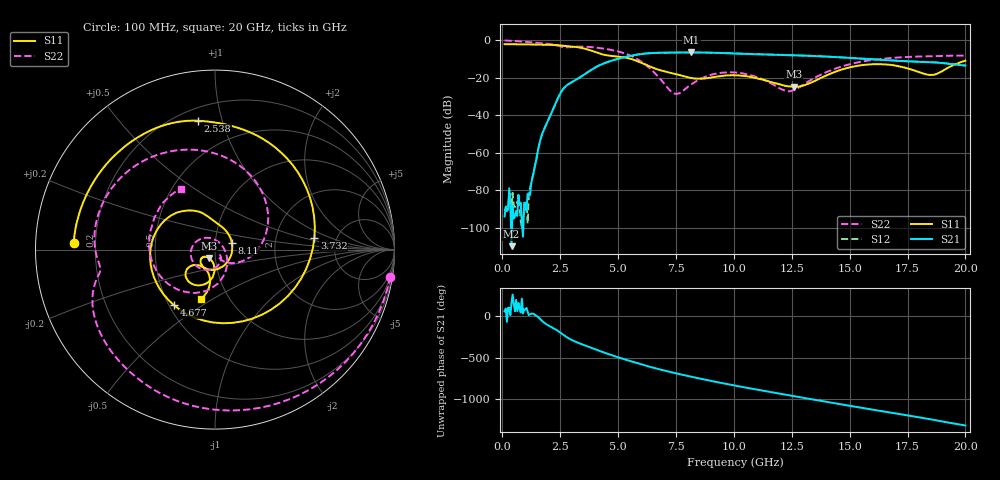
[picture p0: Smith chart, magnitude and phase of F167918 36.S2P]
!  2-Port S-parameters saved by WinCal
! VAR MeasName=S-Parameters (CALIBRATED_DATA) read from VNA (N5242A)
! VAR MeasDate=2016-11-22 10:26:28
! VAR NAME=F167918 36
! VAR FILENAME=F167918 36.S2P
! VAR DATE=2016-11-22 10:26:28
! VAR PHYS_PORTS=1,2
# Hz S DB R 50
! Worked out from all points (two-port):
!   401 points, 100 MHz to 20 GHz, reference 50 ohm
!   highest |S21| = -6.49 dB at 8.159 GHz (marker M1); lowest = -109.7 dB at 398.5 MHz (marker M2)
!   |S21| within 3 dB of the highest: 5.122 GHz to 15.18 GHz (10.06 GHz wide, 99.1 % of centre)
!   lowest |S11| = -24.8 dB at 12.59 GHz (marker M3), VSWR 1.12, Z = 46.6 - j4.41 ohm
!   |S11| at or under -10 dB: 5.578 GHz to end of sweep
!   |S22| runs from -28.6 to -0.1 dB; largest |S21 - S12| = 0.005
!   S11 on the Smith chart (normalised r, x): 100 MHz: 0.12, +0.02; 2.538 GHz: 0.28, +0.84; 3.732 GHz: 3.39, +0.65; 4.677 GHz: 0.53, -0.39; 8.11 GHz: 1.20, +0.09; 20 GHz: 0.74, -0.45
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1e8  -2.07 177.3  -93.89 59.4  -91.08 152.3  -0.10 -8.7
3.985e8  -2.10 169.3  -109.69 158.8  -89.02 177.6  -0.29 -33.0
1.14475e9  -2.23 149.0  -81.51 14.4  -83.80 37.4  -0.96 -87.9
1.74175e9  -2.35 130.4  -49.30 -62.0  -49.34 -62.2  -1.62 -124.9
2.53775e9  -2.80 97.5  -27.63 157.0  -27.63 156.8  -3.42 -166.5
3.43325e9  -4.11 38.5  -19.10 23.2  -19.12 23.2  -3.37 160.8
3.73175e9  -5.07 6.8  -16.65 -8.1  -16.67 -7.9  -3.53 146.4
4.22925e9  -7.19 -61.8  -13.16 -60.5  -13.13 -60.3  -4.18 121.4
4.677e9  -8.29 -126.5  -11.06 -105.0  -10.99 -105.2  -5.08 97.7
5.72175e9  -10.58 135.7  -7.82 163.5  -7.84 163.2  -9.28 30.3
6.7665e9  -15.75 93.7  -6.66 81.8  -6.69 81.6  -19.86 -46.0
7.463e9  -17.95 66.4  -6.55 34.8  -6.57 34.7  -28.51 -56.0
8.10975e9  -19.98 20.9  -6.50 -5.6  -6.51 -5.6  -23.94 -57.8
8.1595e9  -20.09 16.2  -6.49 -8.6  -6.51 -8.7  -23.54 -60.1
1.005e10  -18.64 -119.7  -7.04 -115.8  -7.04 -115.7  -17.17 -165.8
1.129375e10  -21.13 -147.0  -7.56 -179.0  -7.54 -179.0  -21.06 132.3
1.258725e10  -24.79 -125.0  -7.99 117.5  -8.01 117.3  -26.42 15.7
1.338325e10  -22.33 -96.9  -8.34 78.4  -8.32 78.5  -20.74 -42.1
1.49255e10  -14.66 -101.5  -9.34 4.4  -9.29 4.3  -12.97 -98.3
1.67165e10  -13.09 -136.9  -10.65 -79.0  -10.68 -79.1  -9.51 -151.4
1.855725e10  -18.46 -121.4  -11.71 -165.4  -11.68 -165.5  -8.53 160.3
2e10  -10.85 -105.7  -13.49 123.5  -13.36 123.4  -8.21 119.6
